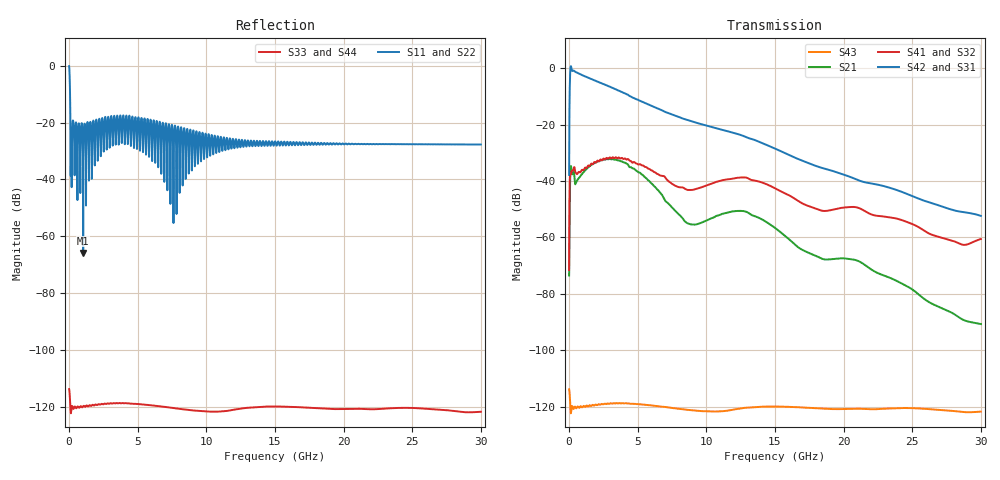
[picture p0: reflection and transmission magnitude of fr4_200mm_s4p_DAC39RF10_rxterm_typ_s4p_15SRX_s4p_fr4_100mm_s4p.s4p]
! Touchstone generated by fitter/viewer
# HZ S  RI R 5.000000e+01
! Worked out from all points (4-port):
!   3899 points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, 7.694 MHz to 30 GHz, reference 50 ohm
!   strongest paths, dB at 7.694 MHz, 7.502 GHz, 15 GHz, 22.51 GHz, 30 GHz:
!     S42: -37.8, -16.4, -28.5, -41.3, -52.4
!     S31: -37.8, -16.5, -28.5, -41.2, -52.3
!     S41: -71.6, -41.0, -42.6, -52.3, -60.5
!     S32: -71.5, -41.1, -42.5, -52.5, -60.5
!     S21: -73.5, -49.4, -56.6, -72.7, -90.7
!     S43: -113.8, -120.4, -119.9, -120.8, -121.7
!   lowest |S11| = -65.9 dB at 1.031 GHz (marker M1), VSWR 1.00, Z = 50 - j0.0272 ohm
!   |S11| at or under -10 dB: 76.76 MHz to end of sweep
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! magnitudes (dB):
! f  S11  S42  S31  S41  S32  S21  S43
! 7.694 MHz  -0.1  -37.8  -37.8  -71.6  -71.5  -73.5  -113.8
! 215.4 MHz  -28.3  -0.8  -0.8  -36.3  -36.4  -37.4  -119.8
! 1.031 GHz  -65.9  -2.6  -2.6  -36.2  -36.3  -37.0  -119.9
! 3.716 GHz  -17.7  -8.2  -8.2  -32.0  -32.0  -32.9  -118.7
! 8.725 GHz  -37.9  -18.5  -18.6  -43.2  -43.2  -55.1  -121.1
! 12.8 GHz  -26.2  -24.2  -24.2  -38.7  -38.7  -50.7  -120.4
! 30 GHz  -27.7  -52.4  -52.3  -60.5  -60.5  -90.7  -121.7
